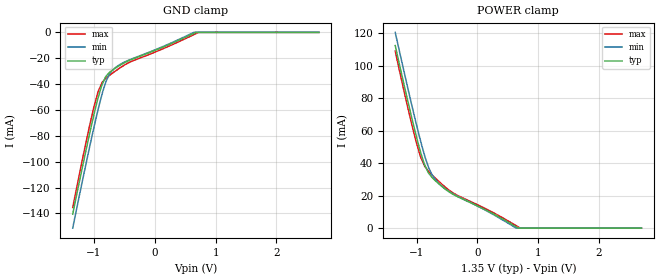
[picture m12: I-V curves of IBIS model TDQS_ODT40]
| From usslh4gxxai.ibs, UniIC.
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| MODEL TDQS_ODT40 (TDQS Terminator Model with 40ohm ODT, 800-2133Mbps)
[Model]   TDQS_ODT40
Model_type   Terminator
|   typ   min   max
|C_comp   0.965pF   0.916pF   1.023pF
C_comp_power_clamp   0.4825pF   0.4580pF   0.5115pF
C_comp_gnd_clamp   0.4825pF   0.4580pF   0.5115pF
| Note: C_comp changes when the ODT circuit is enabled.
[Voltage Range]   1.3500V   1.2830V   1.4250V
[Temperature Range]   45.0   95.0   -40.0
[GND Clamp]
|   Voltage   I(typ)   I(min)   I(max)
-1.35V    -140.6mA   -151.4mA   -135.4mA
-1.075V   -78.79mA   -89.12mA   -72.64mA
-1.005V   -64.28mA   -74.23mA   -58.32mA
-935mV    -51mA      -60.09mA   -46.14mA
-875mV    -41.28mA   -49.01mA   -39.62mA
-800mV    -33.79mA   -37.59mA   -35.32mA
-745mV    -30.93mA   -32.17mA   -33.27mA
-640mV    -27.38mA   -26.98mA   -29.63mA
-400mV    -21.26mA   -20.92mA   -22.77mA
640mV     -769.1uA   -43.13uA   -1.774mA
720mV     0A         0A         0A
2.7V      0A         0A         0A
[POWER Clamp]
|   Voltage   I(typ)   I(min)   I(max)
-1.35V    112.5mA    120.7mA    109.1mA
-1.075V   67.44mA    75.31mA    63.48mA
-935mV    47.05mA    54.01mA    44.1mA
-875mV    39.82mA    45.82mA    38.92mA
-810mV    34.41mA    38.26mA    35.42mA
-750mV    31.45mA    33.22mA    33.03mA
-690mV    29.22mA    29.94mA    30.83mA
-550mV    24.74mA    24.87mA    26.01mA
-340mV    19.7mA     19.9mA     20.47mA
640mV     765.8uA    22.39uA    1.479mA
705mV     0A         0A         0A
2.7V      0A         0A         0A
